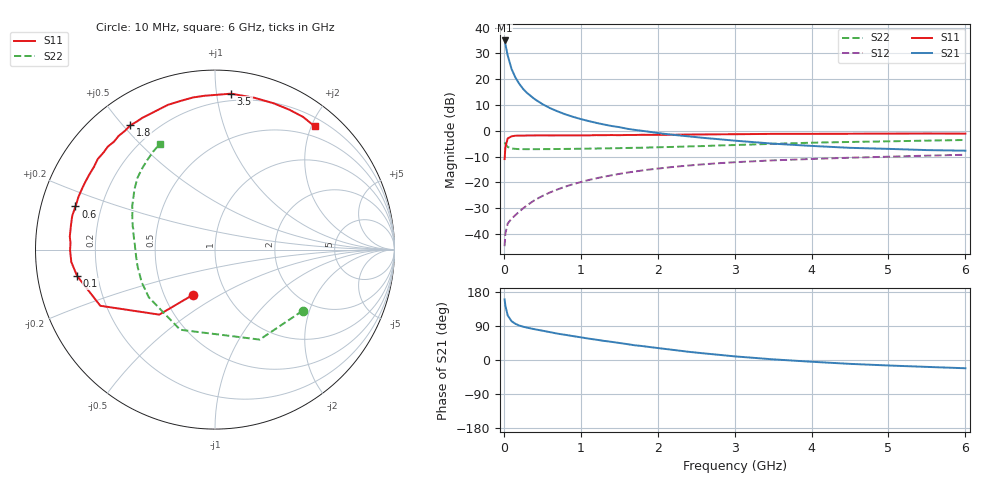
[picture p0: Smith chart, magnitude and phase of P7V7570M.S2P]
! SIEMENS Small Signal Semiconductors
! BFP196
! Si NPN RF Bipolar Junction Transistor in SOT143
! VCE = 0.75 V  IC = 70 mA
! Common Emitter S-Parameters:  May  1996
# GHz  S  MA  R  50
!  f  S11  S21  S12  S22
! GHz  MAG  ANG  MAG  ANG  MAG  ANG  MAG  ANG
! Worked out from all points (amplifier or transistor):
!   36 points, 10 MHz to 6 GHz, reference 50 ohm
!   highest |S21| = 35.0 dB at 10 MHz (marker M1)
!   |S21| within 3 dB of that: start of sweep to 30.86 MHz
!   unconditionally stable (mu >= 1): 225.5 MHz to end of sweep
!   at 250 MHz: K = 1.04, MAG = 21.9 dB, |S12| = -30.1 dB
!   at 1.4 GHz: K = 1.16, MAG = 7.1 dB, |S12| = -17.2 dB
!   at 6 GHz: K = 1.07, MAG = -0.8 dB, |S12| = -9.3 dB
!   S11 on the Smith chart (normalised r, x): 10 MHz: 0.69, -0.38; 100 MHz: 0.12, -0.09; 600 MHz: 0.11, +0.15; 1.8 GHz: 0.11, +0.52; 3.5 GHz: 0.15, +1.10; 6 GHz: 0.33, +2.05
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0.01  0.2828 -116.3  56.54 159.9  0.0058 66.8  0.5955 -34.9
0.02  0.4771 -130.6  48.06 143.3  0.0102 57.7  0.5598 -63.6
0.05  0.7115 -153.9  29 117.7  0.0159 43.8  0.4869 -113.5
0.1  0.7823 -169.2  15.88 102.4  0.0198 43.6  0.4547 -144.2
0.15  0.8037 -175.1  10.83 95.5  0.0232 48.3  0.4471 -156.2
0.2  0.8074 -179.7  8.175 91.0  0.0271 53.2  0.4416 -162.6
0.25  0.8062 177.2  6.514 87.9  0.0314 56.6  0.4415 -167.0
0.3  0.8123 174.9  5.45 85.5  0.0358 59.1  0.4409 -169.6
0.4  0.8141 170.2  4.125 81.2  0.0453 62.0  0.4409 -173.6
0.5  0.8174 166.7  3.308 77.4  0.0544 63.1  0.4416 -176.4
0.6  0.8137 162.8  2.758 73.5  0.0639 63.3  0.4424 -178.4
0.7  0.8154 158.9  2.381 69.5  0.0732 63.1  0.444 179.7
0.8  0.8148 155.8  2.087 66.4  0.0829 62.5  0.4458 178.4
1.1  0.8167 145.7  1.549 56.5  0.111 59.4  0.452 174.1
1.4  0.8281 136.1  1.242 47.9  0.1373 55.0  0.4591 170.5
1.8  0.8379 124.3  1 36.8  0.1704 48.4  0.4699 165.7
2.2  0.8394 113.4  0.837 26.7  0.1996 41.8  0.4876 160.6
2.8  0.8564 98.2  0.687 13.6  0.2358 32.2  0.5207 152.4
3.5  0.8734 84.1  0.564 1.7  0.2675 21.7  0.5599 143.3
4.5  0.8782 68.1  0.468 -10.2  0.301 9.3  0.6082 131.8
5.5  0.8873 56.4  0.423 -18.2  0.33 -1.5  0.646 122.2
6  0.8829 51.1  0.412 -21.8  0.3431 -7.3  0.6642 117.3
